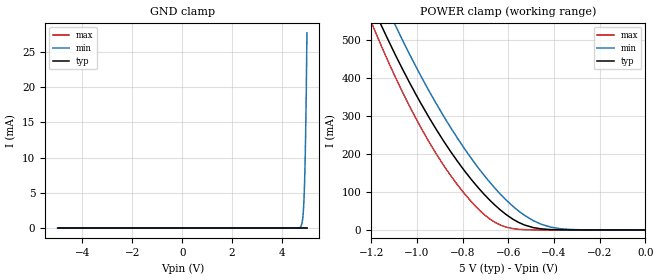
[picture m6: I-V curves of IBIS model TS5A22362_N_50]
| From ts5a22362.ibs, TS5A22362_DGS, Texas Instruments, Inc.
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[Model]   TS5A22362_N_50
Model_type  Terminator
| variable   typ   min   max
C_comp   68.94pF   62.25pF   75.63pF
| C_tri-state   68.94pF   62.25pF   75.63pF
[Temperature Range]   40   100   -40
| Ambient temperature   25   85   -40
[Voltage range]   5   4.5   5.5
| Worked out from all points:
|   POWER clamp passes 1 mA (typ) near -0.41 V on its own axis
[GND Clamp]
| TS5A22362_N_50
|   Voltage   I(typ)   I(min)   I(max)
-5V       -2.185nA   -228.3nA   -316.6pA
4.725V    1.148nA    112.6uA    48.68pA
4.785V    1.166nA    488.8uA    50.46pA
4.83V     1.18nA     1.365mA    51.8pA
4.865V    1.195nA    2.893mA    52.84pA
4.895V    1.219nA    5.282mA    53.73pA
4.91V     1.241nA    7.004mA    54.17pA
4.925V    1.276nA    9.154mA    54.62pA
4.95V     1.399nA    13.82mA    55.36pA
4.975V    1.713nA    19.96mA    56.1pA
4.985V    1.951nA    22.85mA    56.39pA
5V        2.531nA    27.66mA    56.84pA
[POWER Clamp]
| TS5A22362_N_50
|   Voltage   I(typ)   I(min)   I(max)
-5V       11.22A     11.18A     12.52A
-1.185V   578.3mA    659.8mA    527.2mA
-1.155V   538.6mA    619mA      484.7mA
-1.095V   462.8mA    540.7mA    404.2mA
-1.065V   426.8mA    503.3mA    366.3mA
-980mV    331.2mA    403.2mA    267.3mA
-855mV    209.2mA    272.7mA    145.9mA
-760mV    131.8mA    187.2mA    73.44mA
-660mV    66.35mA    111.2mA    20.7mA
-530mV    13.28mA    38.96mA    854.2uA
-415mV    1.069mA    7.67mA     14.98uA
0V        0A         0A         0A
